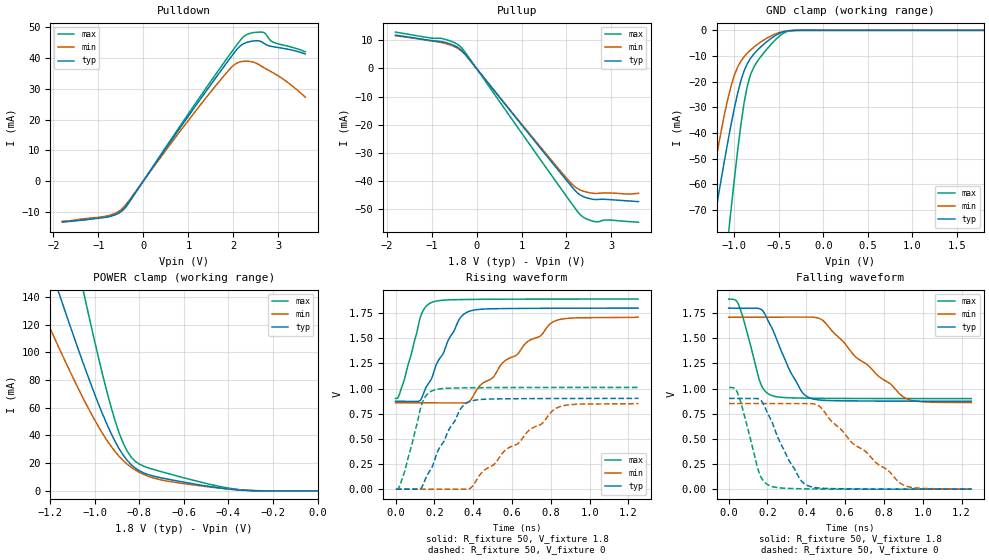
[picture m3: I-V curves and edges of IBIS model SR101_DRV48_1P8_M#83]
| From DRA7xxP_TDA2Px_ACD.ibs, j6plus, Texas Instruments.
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| Model based on original model for DDR_SEIOPB_V
|   Sub model SR101_DRV48_1P8
[model]   SR101_DRV48_1P8_M#83
|[Description]  [1.8V-I/O-X-X]
|   , ,
|[Input Load]
|[Output Drive]
|Voltage   1.8V
|Mode   I/O
Model_type   I/O
Polarity   Non-Inverting
Enable   Active-Low
Vinl =  0.775
Vinh =  1.025
Cref =  15.0000pF
Rref =  100.0000M
Vref =  0V
Vmeas =  0.9
C_comp   2p   2p   2p
[Model Spec]
Vinl   0.78   0.735   0.825
Vinh   1.02   0.975   1.065
[Receiver Thresholds]
Tslew_ac = 0.5n
Vth = 0.9
Vth_max = 0.945
Vth_min = 0.81
Vinh_ac = 0.2
Vinh_dc = 0.125
Vinl_ac = -0.2
Vinl_dc = -0.125
[Temperature Range]   25   125   -40
[Voltage Range]   1.8   1.71   1.89
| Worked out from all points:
|   slope of the pulldown table from 0 to 0.27 V, typ, clamps not added: 46.9 ohm
|   slope of the pullup table from 0 to 0.27 V, typ, clamps not added: 49.7 ohm
|   GND clamp passes 1 mA (typ) near -0.48 V on its own axis
|   POWER clamp passes 1 mA (typ) near -0.38 V on its own axis
|   rising waveform, R_fixture 50, V_fixture 1.8: 20-80 % time 138ps typ, 321ps min, 78.6ps max; typ from 0.874 V to 1.8 V
|   rising waveform, R_fixture 50, V_fixture 0: 20-80 % time 139ps typ, 322ps min, 78.6ps max; typ from 0 V to 0.903 V
|   falling waveform, R_fixture 50, V_fixture 1.8: 20-80 % time 131ps typ, 293ps min, 79.9ps max; typ from 1.8 V to 0.874 V
|   falling waveform, R_fixture 50, V_fixture 0: 20-80 % time 135ps typ, 303ps min, 79.6ps max; typ from 0.903 V to 0 V
[POWER_clamp]
-1.8V     464.6mA    344.4mA    740.8mA
-1.273V   197mA      143.3mA    314.4mA
-1.164V   144mA      104.2mA    229mA
-1.145V   135.3mA    97.86mA    215mA
-1.055V   93.25mA    67.59mA    146.5mA
-1.036V   85.18mA    61.89mA    133.3mA
-909.1mV  35.72mA    28.41mA    50.73mA
-872.7mV  25.87mA    21.94mA    34.5mA
-818.2mV  16.45mA    15.08mA    21.33mA
-690.9mV  9.084mA    7.592mA    13.42mA
-400mV    1.38mA     1.43mA     2.039mA
0V        227.3nA    761nA      1.176uA
[Pulldown]
-1.8V     -13.45mA   -13.11mA   -13.3mA
-818.2mV  -11.81mA   -11.44mA   -11.72mA
-600mV    -10.83mA   -10.36mA   -10.81mA
-436.4mV  -9.068mA   -8.512mA   -9.288mA
1.255V    26.38mA    24.53mA    27.32mA
1.855V    38.53mA    35.35mA    39.84mA
2.073V    42.76mA    38.34mA    44.25mA
2.291V    45.11mA    39mA       47.65mA
2.618V    45.4mA     37.45mA    48.49mA
2.727V    44.4mA     36.48mA    47.76mA
2.891V    43.71mA    35.16mA    45.15mA
3.6V      41.36mA    27.26mA    42.08mA
[Pullup]
-1.8V     11.9mA     11.66mA    12.97mA
-1.036V   10.04mA    9.888mA    10.91mA
-763.6mV  9.523mA    9.186mA    10.68mA
-490.9mV  8.144mA    7.787mA    9.204mA
-327.3mV  6.377mA    6.133mA    7.311mA
2.018V    -40.23mA   -39.43mA   -46mA
2.182V    -43.37mA   -42.12mA   -49.65mA
2.345V    -45.48mA   -43.6mA    -52.72mA
2.509V    -46.4mA    -44.3mA    -54.07mA
2.673V    -46.74mA   -44.55mA   -54.7mA
2.891V    -46.69mA   -44.38mA   -54.01mA
3.6V      -47.48mA   -44.49mA   -54.81mA
[GND_clamp]
-1.8V     -200.8mA   -187.9mA   -345.9mA
-1.327V   -95.75mA   -76.22mA   -171.1mA
-1.255V   -80.19mA   -60.47mA   -144.9mA
-1.218V   -72.53mA   -52.92mA   -131.9mA
-1.073V   -43.32mA   -26.59mA   -81.54mA
-1.036V   -36.61mA   -21.6mA    -69.55mA
-963.6mV  -24.61mA   -14.37mA   -47.01mA
-854.5mV  -12.98mA   -8.864mA   -21.66mA
-781.8mV  -9.263mA   -6.573mA   -14.36mA
-672.7mV  -5.498mA   -3.827mA   -8.897mA
-345.5mV  -48.81uA   -73.08uA   -79.37uA
1.8V      227.3nA    3.986uA    988nA
[Ramp]
dV/dt_f 0.55615029/0.1313763n  0.5115838/0.29384781n 0.59382977/79.895776p
dV/dt_r 0.54252637/0.13947508n 0.51213726/0.32269655n 0.60753124/78.650365p
R_load = 50
[Rising Waveform]
R_fixture = 50
V_fixture = 1.8
V_fixture_min = 1.71
V_fixture_max = 1.89
0s        873.8mV    858.6mV    901.8mV
15.62ps   873.8mV    858.6mV    921.7mV
42.91ps   873.1mV    858.6mV    1.072V
132.1ps   895.3mV    858.6mV    1.733V
186.8ps   1.104V     858.7mV    1.857V
326ps     1.681V     858.1mV    1.885V
381.5ps   1.77V      874.3mV    1.886V
555.7ps   1.795V     1.263V     1.889V
816.8ps   1.798V     1.668V     1.89V
1.25ns    1.8V       1.71V      1.89V
[Rising Waveform]
R_fixture = 50
V_fixture = 0
V_fixture_min = 0
V_fixture_max = 0
1.915ps   0V         0V         0V
18.63ps   0V         0V         21.05mV
45.88ps   0V         0V         168.7mV
136.9ps   24.33mV    0V         855.5mV
191.3ps   232mV      0V         980.1mV
330.6ps   784.5mV    0V         1.007V
388.4ps   874.9mV    13.52mV    1.008V
563ps     898.7mV    382.9mV    1.01V
830ps     901.4mV    806.7mV    1.011V
1.252ns   902.5mV    851.6mV    1.011V
[Falling Waveform]
R_fixture = 50
V_fixture = 1.8
V_fixture_min = 1.71
V_fixture_max = 1.89
0s        1.8V       1.71V      1.89V
49.78ps   1.8V       1.71V      1.84V
161.1ps   1.793V     1.71V      1.067V
217.7ps   1.621V     1.71V      934.4mV
319.3ps   1.162V     1.71V      908.2mV
418.7ps   906.4mV    1.711V     904.4mV
486.2ps   883.8mV    1.677V     903.1mV
651.3ps   877.3mV    1.32V      901.6mV
910.3ps   875mV      905.6mV    900.9mV
1.25ns    873.8mV    858.6mV    900.8mV
[Falling Waveform]
R_fixture = 50
V_fixture = 0
V_fixture_min = 0
V_fixture_max = 0
1.915ps   902.5mV    851.6mV    1.011V
45.17ps   902.7mV    851.6mV    959.9mV
156.2ps   895.8mV    851.6mV    166.1mV
212.1ps   713.1mV    851.6mV    33.76mV
310.3ps   287.2mV    851.4mV    7.215mV
414.4ps   29.8mV     851.8mV    2.851mV
470.7ps   10.57mV    820.2mV    0V
636.9ps   3.055mV    459.7mV    0V
898.4ps   0V         43.14mV    0V
1.252ns   0V         0V         0V
